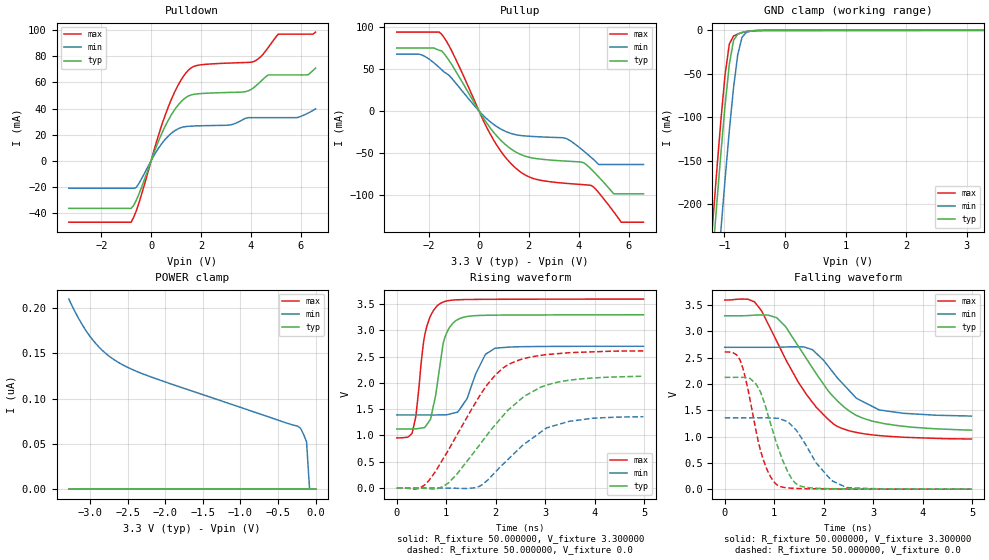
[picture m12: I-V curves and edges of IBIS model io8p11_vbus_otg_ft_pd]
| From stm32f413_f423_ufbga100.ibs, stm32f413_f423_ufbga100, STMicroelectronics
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|   Model io8p11_vbus_otg_ft_pd
[Model]  io8p11_vbus_otg_ft_pd
Model_type I/O
Polarity   Non-Inverting
Enable   Active-Low
Vinl =   0.990000V
Vinh =   2.310000V
Vmeas =  1.650000V
Cref =   30.000000pF
Rref =   100.000000M
Vref =   0.0V
C_comp   3.304800pF   3.199300pF   3.429300pF
[Temperature Range]   25.000000   0.125000k   -40.000000
[Pullup Reference]   3.300000V   2.700000V   3.600000V
[Pulldown Reference]   0.0V   0.0V   0.0V
[POWER Clamp Reference]   3.300000V   2.700000V   3.600000V
[GND Clamp Reference]   0.0V   0.0V   0.0V
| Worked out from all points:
|   slope of the pulldown table from 0 to 0.495 V, typ, clamps not added: 20.9 ohm
|   slope of the pullup table from 0 to 0.495 V, typ, clamps not added: 22.6 ohm
|   GND clamp passes 1 mA (typ) near -0.61 V on its own axis
|   rising waveform, R_fixture 50.000000, V_fixture 3.300000: 20-80 % time 233ps typ, 350ps min, 206ps max; typ from 1.12 V to 3.3 V
|   rising waveform, R_fixture 50.000000, V_fixture 0.0: 20-80 % time 1.17ns typ, 982ps min, 1.02ns max; typ from 0 V to 2.13 V
|   falling waveform, R_fixture 50.000000, V_fixture 3.300000: 20-80 % time 1.03ns typ, 811ps min, 1.01ns max; typ from 3.3 V to 1.12 V
|   falling waveform, R_fixture 50.000000, V_fixture 0.0: 20-80 % time 450ps typ, 585ps min, 371ps max; typ from 2.13 V to 0 V
[Pulldown]
|Voltage   I(typ)   I(min)   I(max)
-3.3V     -36.41mA   -21.08mA   -47.03mA
-800mV    -36.41mA   -21.08mA   -47.03mA
-600mV    -30.48mA   -20.53mA   -38.65mA
700mV     31.4mA     19.11mA    41.71mA
1.2V      45.15mA    25.37mA    61.75mA
1.6V      50.35mA    26.5mA     71.06mA
3.1V      52.27mA    27.26mA    74.75mA
4.1V      55.7mA     32.99mA    75.8mA
4.7V      65.72mA    32.99mA    86.69mA
5.1V      65.72mA    32.99mA    96.9mA
6.3V      65.87mA    36.5mA     96.9mA
6.6V      70.93mA    39.71mA    98.5mA
[Pullup]
|Voltage   I(typ)   I(min)   I(max)
-3.3V     74.73mA    67.41mA    93.65mA
-2.3V     74.73mA    66.57mA    93.65mA
-1.5V     71.37mA    49.01mA    91.08mA
500mV     -22.07mA   -14mA      -30.03mA
1.6V      -50.64mA   -28.81mA   -70.96mA
3.5V      -59.53mA   -32.66mA   -85.92mA
4.2V      -61.44mA   -47.48mA   -87.46mA
4.5V      -69.06mA   -55.13mA   -88.4mA
4.8V      -78.23mA   -63.5mA    -96.84mA
5.4V      -98.3mA    -63.5mA    -119.6mA
5.7V      -98.3mA    -63.5mA    -132mA
6.6V      -98.3mA    -63.5mA    -132mA
[GND_clamp]
|Voltage   I(typ)   I(min)   I(max)
-3.3V     -2.318A    -2.397A    -2.291A
-1.2V     -265.6mA   -356.2mA   -227.3mA
-1.13V    -202.8mA   -293mA     -164.3mA
-1.06V    -142.3mA   -231.2mA   -104.3mA
-990mV    -86.15mA   -171.7mA   -51.01mA
-920mV    -39.05mA   -115.6mA   -15.73mA
-850mV    -11.41mA   -65.74mA   -6.38mA
-780mV    -4.058mA   -27.6mA    -4.167mA
-710mV    -2.296mA   -7.89mA    -2.605mA
-640mV    -1.302mA   -2.283mA   -1.381mA
-570mV    -629.1uA   -918.9uA   -580.8uA
3.28V     81.28uA    57.87uA    93.98uA
[POWER_clamp]
|Voltage   I(typ)   I(min)   I(max)
-3.28V    0A         210.1nA    0A
-3.12V    0A         184.2nA    0A
-2.96V    0A         164.6nA    0A
-2.8V     0A         150.7nA    0A
-2.6V     0A         139nA      0A
-2.16V    0A         123.2nA    0A
-240mV    0A         69.7nA     0A
-200mV    0A         67.32nA    0A
-160mV    0A         60.72nA    0A
-120mV    0A         52.23nA    0A
-80mV     0A         0A         0A
0V        0A         0A         0A
[Ramp]
| variable   typ   min   max
dV/dt_r  1.25886/1.15667n   0.80034/0.97034n   1.55964/1.01751n
dV/dt_f  1.27482/1.00952n   0.76698/0.78353n   1.56901/1.00615n
R_load = 50.000000
[Rising Waveform]
R_fixture= 50.000000
V_fixture= 3.300000
V_fixture_min= 2.700000
V_fixture_max= 3.600000
|time   V(typ)   V(min)   V(max)
0s        1.123V     1.391V     954mV
310.3ps   1.125V     1.391V     1.043V
390.4ps   1.127V     1.391V     1.404V
570.6ps   1.16V      1.391V     2.937V
680.7ps   1.306V     1.39V      3.274V
880.9ps   2.393V     1.392V     3.514V
961ps     2.835V     1.393V     3.549V
1.131ns   3.137V     1.422V     3.578V
1.992ns   3.291V     2.663V     3.593V
4.985ns   3.299V     2.699V     3.598V
[Rising Waveform]
R_fixture= 50.000000
V_fixture= 0.0
V_fixture_min= 0.0
V_fixture_max= 0.0
|time   V(typ)   V(min)   V(max)
0s        345.3uV    194.5uV    641.5uV
560.6ps   -7.069mV   182.9uV    54.55mV
951ps     36.36mV    -1.04mV    577.9mV
1.662ns   806.9mV    26.93mV    1.736V
1.992ns   1.206V     303.5mV    2.152V
2.242ns   1.478V     538.9mV    2.343V
2.583ns   1.751V     841.2mV    2.467V
3.033ns   1.959V     1.147V     2.541V
3.964ns   2.095V     1.329V     2.593V
4.985ns   2.127V     1.357V     2.611V
[Falling Waveform]
R_fixture= 50.000000
V_fixture= 3.300000
V_fixture_min= 2.700000
V_fixture_max= 3.600000
|time   V(typ)   V(min)   V(max)
0s        3.299V     2.699V     3.598V
600.6ps   3.31V      2.699V     3.565V
750.8ps   3.314V     2.699V     3.382V
1.051ns   3.262V     2.7V       2.815V
1.481ns   2.728V     2.708V     2.044V
1.772ns   2.309V     2.654V     1.654V
2.252ns   1.704V     2.146V     1.207V
2.663ns   1.403V     1.728V     1.079V
3.123ns   1.266V     1.507V     1.02V
4.985ns   1.123V     1.391V     954mV
[Falling Waveform]
R_fixture= 50.000000
V_fixture= 0.0
V_fixture_min= 0.0
V_fixture_max= 0.0
|time   V(typ)   V(min)   V(max)
0s        2.127V     1.357V     2.611V
310.3ps   2.128V     1.357V     2.456V
460.5ps   2.116V     1.357V     1.946V
620.6ps   2.014V     1.357V     1.169V
840.8ps   1.521V     1.359V     404.3mV
1.081ns   784.6mV    1.348V     69.49mV
1.471ns   85.7mV     1.09V      13.82mV
2.152ns   9.937mV    170.9mV    4.286mV
2.462ns   6.127mV    30.92mV    3.22mV
4.985ns   345.3uV    194.5uV    641.5uV
